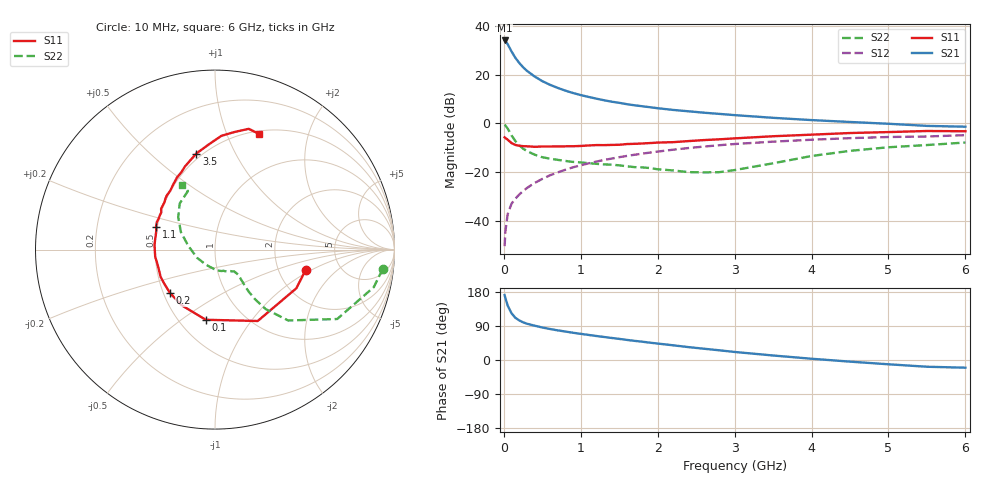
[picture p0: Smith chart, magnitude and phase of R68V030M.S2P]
! SIEMENS Small Signal Semiconductors
! BFR193
! Si NPN RF Bipolar Junction Transistor in SOT23
! VCE = 8 V  IC = 30 mA
! Common Emitter S-Parameters:  May  1996
# GHz  S  MA  R  50
!  f  S11  S21  S12  S22
! GHz  MAG  ANG  MAG  ANG  MAG  ANG  MAG  ANG
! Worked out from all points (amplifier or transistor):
!   36 points, 10 MHz to 6 GHz, reference 50 ohm
!   highest |S21| = 34.1 dB at 10 MHz (marker M1)
!   |S21| within 3 dB of that: start of sweep to 74.43 MHz
!   unconditionally stable (mu >= 1): 518.8 MHz to 2.194 GHz
!   at 250 MHz: K = 0.88, MSG = 25.4 dB, |S12| = -27.8 dB
!   at 1.4 GHz: K = 1.03, MAG = 10.7 dB, |S12| = -14.5 dB
!   at 6 GHz: K = 0.94, MSG = 1.7 dB, |S12| = -4.8 dB
!   lowest NFmin = 1.90 dB at 450 MHz
!   S11 on the Smith chart (normalised r, x): 10 MHz: 2.83, -0.89; 100 MHz: 0.67, -0.62; 200 MHz: 0.54, -0.30; 1.1 GHz: 0.49, +0.14; 3.5 GHz: 0.47, +0.71; 6 GHz: 0.53, +1.31
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0.01  0.5174 -12.8  50.73 171.3  0.003 82.1  0.9408 -6.6
0.02  0.5019 -25.4  49.37 163.4  0.006 77.7  0.9091 -13.3
0.05  0.4636 -59.1  42.42 143.7  0.0137 70.0  0.783 -29.6
0.1  0.3943 -97.5  30.17 123.3  0.0224 64.9  0.5675 -44.1
0.15  0.3615 -120.9  22.32 111.4  0.0284 64.2  0.4347 -49.6
0.2  0.3484 -135.8  17.54 104.5  0.0345 66.5  0.3551 -51.1
0.25  0.3407 -146.1  14.29 99.4  0.0408 67.2  0.3029 -51.3
0.3  0.3389 -153.4  12.07 95.8  0.047 68.6  0.2707 -50.8
0.4  0.3306 -165.2  9.212 90.5  0.0598 70.4  0.2277 -49.2
0.5  0.3355 -173.1  7.397 85.8  0.0724 71.0  0.2019 -47.9
0.6  0.3354 -179.0  6.222 81.8  0.0859 70.6  0.1885 -47.5
0.8  0.3383 170.5  4.719 75.1  0.1117 69.3  0.1694 -48.3
0.9  0.3398 166.2  4.214 71.9  0.1254 68.7  0.1619 -48.7
1.1  0.3523 158.9  3.506 66.2  0.1509 66.8  0.1531 -52.4
1.3  0.3581 151.6  2.998 60.8  0.1771 64.3  0.1442 -56.4
1.6  0.3766 142.9  2.485 53.0  0.2149 60.5  0.1316 -65.7
2.2  0.4122 127.2  1.894 38.8  0.2883 52.2  0.1081 -93.1
2.8  0.4713 113.3  1.571 25.6  0.3562 43.3  0.0995 -140.3
3.5  0.5453 101.0  1.304 11.9  0.422 32.5  0.1516 171.5
4.5  0.6348 86.8  1.071 -4.3  0.4981 18.6  0.2732 138.6
5.5  0.6985 74.4  0.89 -17.8  0.5386 4.7  0.3595 114.8
6  0.6903 69.3  0.856 -20.3  0.5738 0.9  0.4049 116.9
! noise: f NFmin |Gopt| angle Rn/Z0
0.45  1.9  0.4  180  0.09
0.9  1.95  0.43  -173  0.11
1.8  2.4  0.58  -144  0.24
